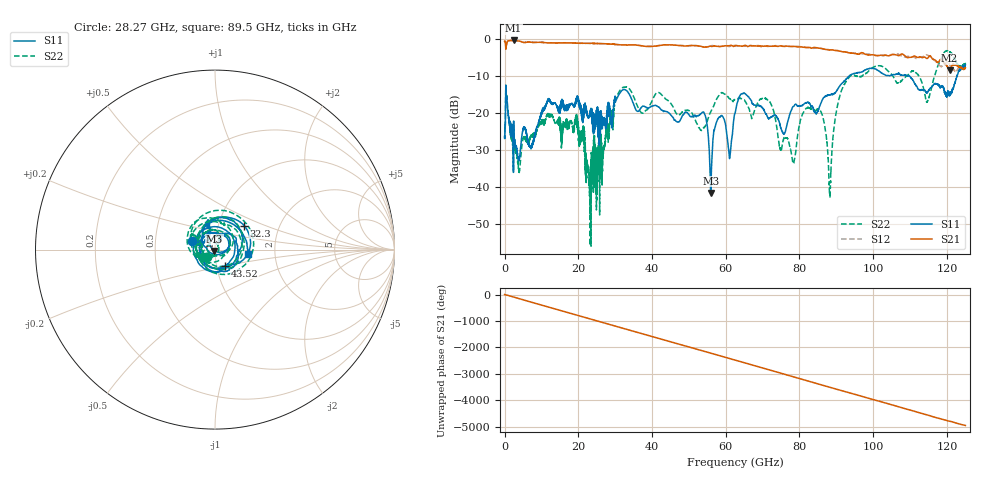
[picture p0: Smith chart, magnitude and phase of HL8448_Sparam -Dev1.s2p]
! 7/28/2025 10:37:03 AM
! H:\PROTOTYPE_DATA\110GHZ - KELVIN BT\7-28-25\3602.S2P
! CHANNEL.1
! TR.MEASUREMENT
! CORRECTED.DATA
! RF.CORRECTION: FULL.TWO.PORT.CAL.PORT.1.2
! AVERAGING: 1 PointByPoint
! IF.BANDWIDTH: 1KHZ
! SWEEPTYPE:  FREQ.SWEEP(Linear)
! Reference Plane Port Info
! PORT:  PORT1  PORT2
! DISTANCE:  0  m  0  m
! TIME:  0  s  0  s
! PHASE.OFFSET:  0 °  0 °
! LOSS:  0  dB  0  dB
! REF.LOSS:  0  dB  0  dB
! REF.FREQ:  0  Hz  0  Hz
! Power Info
! POWER:  -10  dBm  -10  dBm
! EFF.POWER:  -10  dBm  -10  dBm
! POWER(>54G):  -10  dBm  -10  dBm
! EFF.POWER(>54G):  -10  dBm  -10  dBm
! SOURCE.ATTEN:  0  dB  0  dB
! TEST.ATTEN:  0  dB  0  dB
# GHZ S RI R 50.0
! FREQ.GHZ  S11RE  S11IM  S21RE  S21IM  S12RE  S12IM  S22RE  S22IM
!; PortSelection: Port_12
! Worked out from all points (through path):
!   5000 points, 25 MHz to 125 GHz, reference 50 ohm
!   highest |S21| = -0.31 dB at 2.45 GHz (marker M1); lowest = -8.4 dB at 120.7 GHz (marker M2)
!   group delay of S21, straight-line fit = 110 ps
!   lowest |S11| = -41.6 dB at 55.92 GHz (marker M3), VSWR 1.02, Z = 49.6 - j0.706 ohm
!   |S11| at or under -10 dB: start of sweep to 93.37 GHz; 109.898 GHz to 109.9094 GHz (11.36 MHz wide, 0.0103 % of centre); 109.9 GHz to 122.7 GHz (12.74 GHz wide, 11 % of centre)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
!   |S22| runs from -55.9 to -3.0 dB; largest |S21 - S12| = 0.11
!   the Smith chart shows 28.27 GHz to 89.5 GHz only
!   S11 on the Smith chart (normalised r, x): 28.27 GHz: 0.77, +0.07; 32.3 GHz: 1.33, +0.37; 43.52 GHz: 1.10, -0.20; 89.5 GHz: 1.45, -0.08
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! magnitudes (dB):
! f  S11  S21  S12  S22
! 25 MHz  -26.2  -0.5  -0.5  -26.2
! 2.45 GHz  -24.1  -0.3  -0.3  -22.9
! 20.88 GHz  -20.5  -1.1  -1.0  -25.2
! 23.1 GHz  -20.3  -1.1  -1.1  -38.1
! 28.27 GHz  -17.4  -1.2  -1.2  -24.1
! 32.3 GHz  -13.6  -1.5  -1.5  -12.9
! 41.7 GHz  -18.2  -1.7  -1.8  -14.4
! 43.52 GHz  -19.5  -1.5  -1.5  -16.0
! 54.02 GHz  -19.8  -2.1  -2.0  -23.8
! 55.92 GHz  -41.6  -1.9  -1.8  -19.6
! 62.52 GHz  -20.0  -1.7  -1.8  -16.2
! 71.53 GHz  -21.3  -1.8  -1.9  -16.5
! 78.35 GHz  -18.1  -1.9  -1.9  -33.5
! 83.35 GHz  -18.1  -2.4  -2.4  -18.8
! 86.25 GHz  -16.3  -2.5  -2.5  -20.7
! 88.2 GHz  -15.0  -2.9  -2.9  -41.4
! 89.5 GHz  -14.6  -3.0  -3.0  -22.6
! 93.65 GHz  -9.7  -3.7  -3.7  -10.0
! 104.2 GHz  -9.8  -4.4  -4.4  -8.7
! 114.7 GHz  -14.2  -5.1  -4.2  -16.8
! 120.7 GHz  -14.9  -8.4  -6.8  -3.5
! 125 GHz  -6.8  -7.7  -8.2  -6.6
